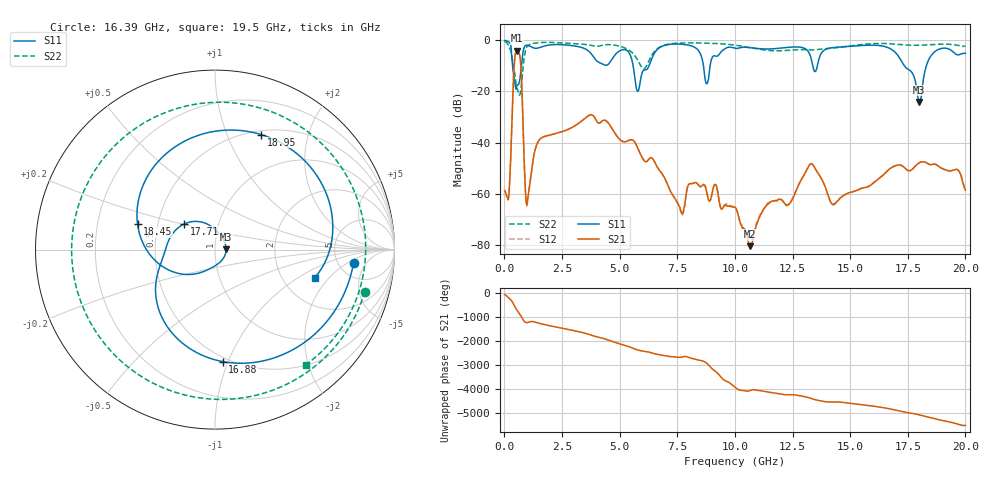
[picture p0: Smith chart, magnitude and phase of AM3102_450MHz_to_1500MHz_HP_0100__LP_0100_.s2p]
!Agilent Technologies,E8364B,MY43040894,A.07.50.67
!Agilent E8364B: A.07.50.67
!Date: Thursday, January 11, 2018 05:36:12
!Correction: S11(Full 2 Port(1,2))
!S21(Full 2 Port(1,2))
!S12(Full 2 Port(1,2))
!S22(Full 2 Port(1,2))
!S2P File: Measurements: S11, S21, S12, S22:
# Hz S  dB  R 50
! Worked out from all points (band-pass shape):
!   1601 points, 10 MHz to 20 GHz, reference 50 ohm
!   highest |S21| = -4.02 dB at 547.2 MHz (marker M1); lowest = -80.5 dB at 10.65 GHz (marker M2)
!   |S21| within 3 dB of the highest: 452.3 MHz to 685.5 MHz (233.2 MHz wide, 41 % of centre)
!   lowest |S11| = -24.1 dB at 18 GHz (marker M3), VSWR 1.13, Z = 56.6 + j0.0704 ohm
!   |S11| at or under -10 dB: 354.8 MHz to 739.8 MHz (384.9 MHz wide, 70.3 % of centre); 5.586 GHz to 6.272 GHz (686.4 MHz wide, 11.6 % of centre); 17.35 GHz to 18.3 GHz (949.7 MHz wide, 5.33 % of centre)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
!   |S22| runs from -21.4 to -0.4 dB; largest |S21 - S12| = 0.0044
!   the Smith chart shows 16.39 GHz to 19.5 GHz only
!   S11 on the Smith chart (normalised r, x): 16.39 GHz: 6.97, -2.53; 16.88 GHz: 0.47, -0.95; 17.71 GHz: 0.68, +0.21; 18.45 GHz: 0.38, +0.14; 18.95 GHz: 0.54, +1.33; 19.5 GHz: 3.00, -1.41
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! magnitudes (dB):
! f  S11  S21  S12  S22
! 10 MHz  -0.1  -58.7  -59.0  -0.4
! 197.4 MHz  -0.7  -60.3  -59.7  -2.7
! 547.2 MHz  -17.8  -4.0  -4.0  -18.9
! 997 MHz  -2.0  -63.5  -63.3  -2.3
! 1.509 GHz  -2.9  -39.0  -39.0  -0.9
! 3.346 GHz  -2.8  -31.6  -31.6  -1.5
! 5.782 GHz  -19.9  -42.1  -42.1  -7.7
! 6.682 GHz  -3.2  -50.3  -50.3  -3.0
! 8.781 GHz  -17.0  -59.3  -59.5  -1.1
! 10.01 GHz  -3.1  -65.2  -65.3  -1.9
! 10.65 GHz  -2.9  -80.5  -79.6  -2.8
! 13.34 GHz  -8.4  -48.3  -48.4  -3.8
! 14.27 GHz  -2.8  -64.0  -64.3  -3.0
! 16.39 GHz  -2.2  -53.0  -52.9  -1.2
! 16.68 GHz  -3.0  -50.5  -50.5  -1.3
! 16.88 GHz  -4.1  -49.4  -49.4  -1.5
! 17.71 GHz  -13.0  -50.2  -50.3  -1.9
! 18 GHz  -24.1  -47.8  -47.9  -1.9
! 18.45 GHz  -6.9  -48.6  -48.5  -1.8
! 18.95 GHz  -3.2  -49.9  -49.9  -1.5
! 19.5 GHz  -4.8  -50.7  -50.6  -1.8
! 20 GHz  -5.1  -58.5  -58.8  -2.4
